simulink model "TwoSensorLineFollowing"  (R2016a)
settings: Solver=FixedStepAuto  StartTime=0.0  StopTime=inf  RelTol=1e-3
libraries: miniQ x2

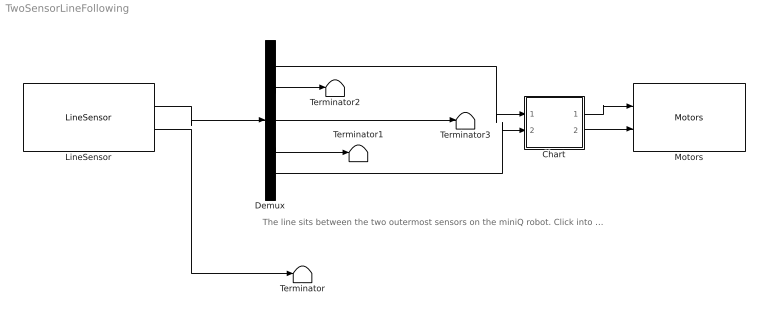
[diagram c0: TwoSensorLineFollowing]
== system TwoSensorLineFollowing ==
  note: The line sits between the two outermost sensors on the miniQ robot. Click into the chart to view how these two sensors allow the robot to stay ontop of a line
  Chart : Stateflow chart  TreatAsAtomicUnit=on
  Demux : Demux  Outputs=5
  LineSensor : miniQ/LineSensor  sampleTime_dd=0.01  maxRawSensors=[800,900,900,900,800]  minRawSensors=[200,280,300,300,220]  debug_dd=off
  Motors : miniQ/Motors  flipLeft=off  flipRight=off
  Terminator{,1..3} (4 alike) : Terminator
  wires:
  LineSensor/2 -> Terminator/1
  LineSensor/1 -> Demux/1
  Demux/3 -> Terminator3/1
  Chart/1(l) -> Motors/1
  Chart/2(r) -> Motors/2
  Demux/2 -> Terminator2/1
  Demux/1 -> Chart/1(ls)
  Demux/4 -> Terminator1/1
  Demux/5 -> Chart/2(rs)

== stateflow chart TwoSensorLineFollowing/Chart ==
  state Forward
    entry: r=50
    l=50
  state If the left sensor detects the line [group]
    the robot turns right.
  state LeftPivot
    entry: r=-150
    l=150
  state RightPivot
    entry: r=150
    l=-150
  state If the right sensor detects the line the robot [group]
    turns left
  (default) -> Forward
  LeftPivot -> Forward : [rs>500]
  RightPivot -> Forward : [ls>500]
  Forward -> LeftPivot : [rs<500]
  Forward -> RightPivot : [ls<500]
  data: ls input; rs input; l output; r output
